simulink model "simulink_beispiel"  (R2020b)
settings: Solver=VariableStepAuto  StartTime=0.0  StopTime=10.0  RelTol=1e-3

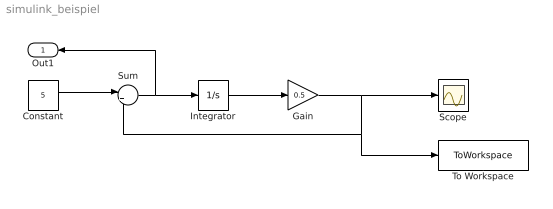
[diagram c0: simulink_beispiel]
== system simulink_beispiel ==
  Constant : Constant  Value=5
  Gain : Gain  Gain=0.5
  Integrator : Integrator
  Scope : Scope
  Sum : Sum  Inputs=|+-
  To Workspace : ToWorkspace  VariableName=simout  SaveFormat=Timeseries  SampleTime=-1
  Out1 : Outport
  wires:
  Constant/1 -> Sum/1
  Sum/1 -> Out1/1, Integrator/1
  Integrator/1 -> Gain/1
  Gain/1 -> To Workspace/1, Sum/2, Scope/1
